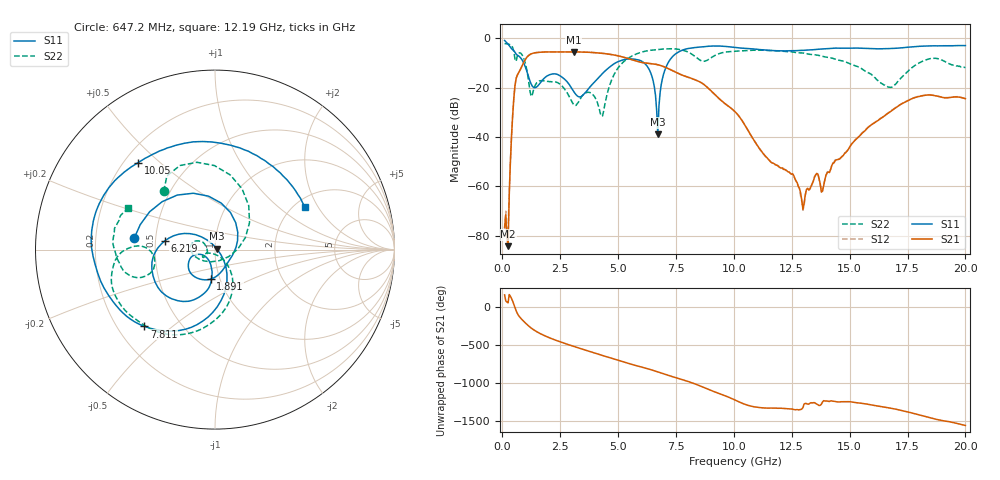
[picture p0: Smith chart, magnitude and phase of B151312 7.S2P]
!  2-Port S-parameters saved by WinCal
! VAR MeasName=S-Parameters (CALIBRATED_DATA) read from VNA (N5244A)
! VAR MeasDate=12/8/2015 5:44:14 PM
! VAR NAME=B151312 7
! VAR FILENAME=B151312 7.S2P
! VAR DATE=12/8/2015 5:44:14 PM
! VAR PHYS_PORTS=1,2
# Hz S DB R 50
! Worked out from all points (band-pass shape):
!   401 points, 100 MHz to 20 GHz, reference 50 ohm
!   highest |S21| = -5.53 dB at 3.085 GHz (marker M1); lowest = -84.3 dB at 249.2 MHz (marker M2)
!   |S21| within 3 dB of the highest: 1.002 GHz to 5.538 GHz (4.536 GHz wide, 139 % of centre)
!   lowest |S11| = -38.9 dB at 6.717 GHz (marker M3), VSWR 1.02, Z = 51.1 + j0.442 ohm
!   |S11| at or under -10 dB: 922.9 MHz to 4.892 GHz (3.969 GHz wide, 137 % of centre); 6.126 GHz to 7.159 GHz (1.033 GHz wide, 15.6 % of centre)
!   |S22| runs from -31.6 to -2.2 dB; largest |S21 - S12| = 0.0014
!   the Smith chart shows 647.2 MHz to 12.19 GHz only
!   S11 on the Smith chart (normalised r, x): 647.2 MHz: 0.38, +0.06; 1.891 GHz: 0.90, -0.31; 6.219 GHz: 0.56, +0.06; 7.811 GHz: 0.31, -0.40; 10.05 GHz: 0.26, +0.43; 12.19 GHz: 2.25, +1.56
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1e8  -0.90 -41.8  -76.58 156.8  -77.36 101.4  -2.19 169.3
2.4925e8  -2.42 -93.0  -84.31 52.2  -78.34 77.2  -2.36 152.1
4.98e8  -5.06 -157.6  -24.36 34.0  -24.35 33.9  -5.36 109.2
6.4725e8  -6.85 171.7  -15.01 -86.8  -15.01 -86.8  -7.28 131.4
1.24425e9  -18.51 7.1  -6.36 80.4  -6.36 80.4  -23.58 -68.4
1.891e9  -15.58 -98.6  -5.57 -30.3  -5.57 -30.3  -17.38 168.0
3.085e9  -21.61 -161.2  -5.53 -162.4  -5.53 -162.4  -27.00 178.0
3.43325e9  -23.48 -123.5  -5.60 163.4  -5.59 163.4  -23.58 -146.3
4.32875e9  -14.27 -97.6  -6.12 77.6  -6.12 77.6  -31.50 -89.0
4.92575e9  -9.83 -116.9  -6.98 20.9  -6.98 20.9  -13.08 -63.0
6.21925e9  -10.90 170.3  -10.07 -91.9  -10.09 -92.0  -5.16 -122.8
6.71675e9  -38.88 22.3  -10.74 -138.8  -10.75 -138.8  -4.61 -139.1
6.7665e9  -27.43 -40.3  -10.86 -143.9  -10.88 -143.8  -4.54 -140.4
7.11475e9  -10.82 -83.5  -12.09 -179.0  -12.06 -179.0  -4.30 -150.3
7.81125e9  -4.72 -132.6  -15.12 115.7  -15.08 115.4  -4.92 -172.1
1.005e10  -3.78 131.5  -29.78 -149.8  -29.84 -149.9  -5.25 -174.2
1.218925e10  -5.11 25.6  -53.17 98.7  -53.22 99.2  -5.37 154.6
1.298525e10  -4.89 -15.1  -69.41 111.3  -69.74 119.7  -6.01 143.8
1.338325e10  -4.69 -32.2  -58.91 172.0  -59.13 175.4  -6.65 138.1
1.67165e10  -4.21 -111.3  -30.08 105.8  -29.92 105.6  -19.88 155.4
1.8408e10  -3.12 -130.7  -23.01 -18.8  -22.94 -18.8  -8.44 164.8
2e10  -2.97 -146.9  -24.51 -125.1  -24.53 -126.3  -11.97 124.1
